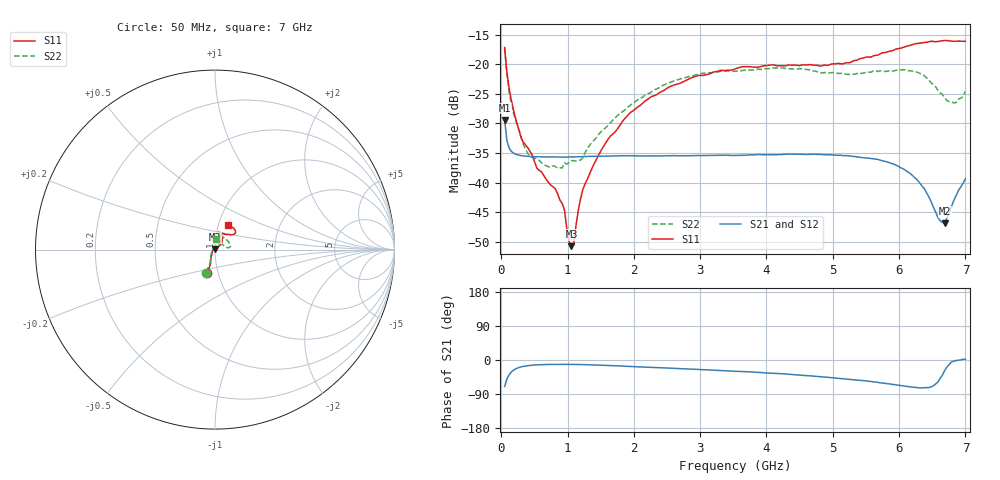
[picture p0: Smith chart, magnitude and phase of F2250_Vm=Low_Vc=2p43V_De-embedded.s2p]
! Integrated Device Technology
! Corporate Headquarters
! 6024 Silver Creek Valley Road
! San Jose, CA 95138  USA
! Phone:  1-408-284-8200
! Toll Free:  1-800-223-1366
! Webpage:  http://www.idt.com/
! Timing and RF Division
! 515 Groton Road, Suite 102
! Westford, MA 01886-6024
! Device:  F2250
! Description: Voltage Variable RF Attenuator
! Frequency:  50.0 -  6000.00 MHz
! Package:  3x3 mm Thin QFN Plastic Package: 16 pin
! Ports:  2 RF, 3 DC
!  Pin  1  = GND
!  Pin  2  = NC
!  Pin  3  = RF1  = Port 1
!  Pin  4  = NC
!  Pin  5  = GND
!  Pin  6  = GND
!  Pin  7  = GND
!  Pin  8  = GND
!  Pin  9  = NC
!  Pin 10  = RF2  = Port 2
!  Pin 11  = NC
!  Pin 12  = GND
!  Pin 13  = GND
!  Pin 14  = VCNTRL
!  Pin 15  = VDD
!  Pin 16  = VMODE
! Vcntrl:  2.430 Volts
! Vmode:  +0.000 Volts
! Vdd:  +3.30  Volts
! Current:  1.176 mA
! Data:  The device was measured on a the F2250 evaluation board which has
!  individual transmission lines to the RF pins.  Data was collected
!  using a calibrated network analyzer.  The evaluation board was
!  de-embedded using a TRL calibration technique.
!  The reference plane is the edge of the package pin.
! Misc:  SN 10
!  Action Tracker AT0258
! Date Measured:  2014-11-26
! Date:  2015-10-15  MJV
! Note:
!  Integrated Device Technology supplies this data as a sample of measured
!  data at the package pin for this product.  Your particular data for this
!  product may vary.
!  Data was taken at 25 degrees C.
!  Integrated Device Technology reserves the right to change this data at anytime.
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# GHz S dB R 50
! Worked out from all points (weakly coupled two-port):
!   201 points, 50 MHz to 7 GHz, reference 50 ohm
!   highest |S21| = -29.41 dB at 50 MHz (marker M1); lowest = -46.9 dB at 6.687 GHz (marker M2)
!   lowest |S11| = -50.7 dB at 1.058 GHz (marker M3), VSWR 1.01, Z = 49.8 + j0.243 ohm
!   |S11| at or under -10 dB: start of sweep to end of sweep
!   |S22| runs from -37.5 to -17.3 dB; largest |S21 - S12| = 6.4e-05
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0.05  -17.18 -108.6  -29.41 -69.8  -29.41 -69.8  -17.27 -111.0
0.08475  -21.45 -107.5  -32.92 -50.4  -32.92 -50.3  -21.75 -110.2
0.15425  -26.23 -116.6  -34.76 -31.2  -34.76 -31.1  -26.82 -122.4
0.29325  -32.22 -127.8  -35.43 -18.5  -35.43 -18.5  -32.10 -137.4
0.3975  -34.08 -141.7  -35.56 -15.0  -35.56 -15.0  -35.04 -160.4
0.91875  -43.53 157.9  -35.69 -11.5  -35.68 -11.5  -37.52 133.5
0.9535  -44.67 169.8  -35.68 -11.5  -35.68 -11.5  -36.66 131.1
1.023  -50.02 144.3  -35.67 -11.6  -35.67 -11.6  -36.62 116.0
1.05775  -50.74 122.9  -35.67 -11.6  -35.67 -11.6  -36.29 110.8
1.0925  -50.34 90.9  -35.66 -11.7  -35.66 -11.7  -36.29 106.3
1.162  -44.66 56.8  -35.64 -11.9  -35.64 -11.9  -36.23 95.6
1.2315  -41.11 44.6  -35.60 -12.1  -35.61 -12.1  -35.78 85.9
1.61375  -32.61 40.9  -35.52 -14.4  -35.52 -14.5  -30.29 65.6
1.9265  -28.40 41.4  -35.47 -16.9  -35.47 -16.9  -27.09 56.7
2.37825  -24.87 47.3  -35.48 -20.3  -35.48 -20.3  -23.99 56.9
3.525  -20.80 72.4  -35.41 -29.5  -35.41 -29.5  -21.19 74.8
4.7065  -20.17 72.3  -35.21 -42.5  -35.20 -42.5  -21.15 72.3
5.85325  -17.81 40.5  -36.63 -63.2  -36.64 -63.3  -21.13 23.0
6.27025  -16.50 40.1  -39.49 -72.5  -39.51 -72.6  -21.35 9.6
6.68725  -15.99 48.8  -46.86 -27.7  -46.83 -27.4  -25.64 28.4
6.861  -16.13 55.1  -42.17 -1.3  -42.13 -1.2  -26.47 58.0
7  -16.12 63.2  -39.35 1.9  -39.30 1.8  -24.62 83.1
